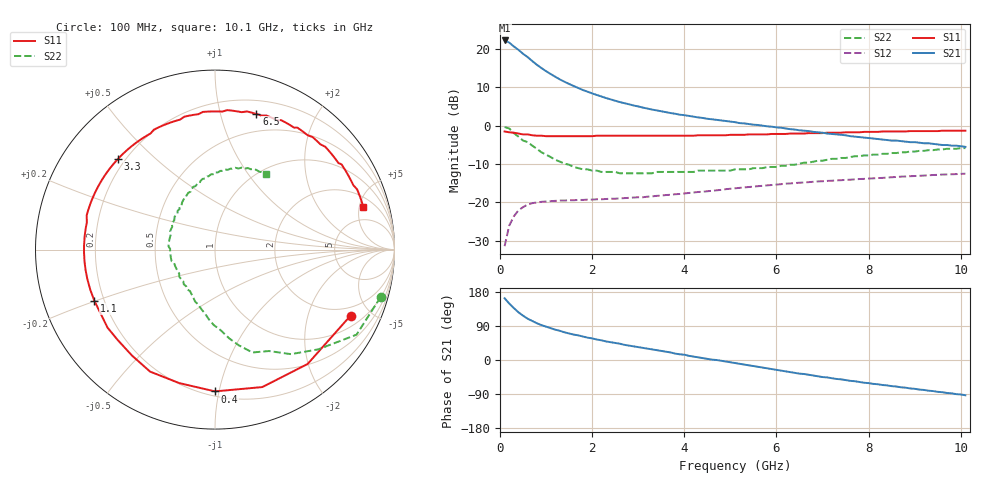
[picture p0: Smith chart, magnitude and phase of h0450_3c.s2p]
!HBFP-0450
!S and NOISE PARAMETERS at Vce=3V  Ic=5mA.  LAST UPDATED  09-04-98
# GHZ S MA R  50
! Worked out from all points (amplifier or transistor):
!   101 points, 100 MHz to 10.1 GHz, reference 50 ohm
!   highest |S21| = 22.2 dB at 100 MHz (marker M1)
!   |S21| within 3 dB of that: start of sweep to 454.6 MHz
!   unconditionally stable (mu >= 1): 2.917 GHz to end of sweep
!   at 1.7 GHz: K = 0.62, MSG = 14.6 dB, |S12| = -19.3 dB
!   at 5.1 GHz: K = 1.23, MAG = 5.7 dB, |S12| = -16.3 dB
!   at 10.1 GHz: K = 1.12, MAG = 1.4 dB, |S12| = -12.5 dB
!   lowest NFmin = 1.14 dB at 1.8 GHz
!   S11 on the Smith chart (normalised r, x): 100 MHz: 1.50, -3.76; 400 MHz: 0.23, -0.97; 1.1 GHz: 0.16, -0.20; 3.3 GHz: 0.17, +0.38; 6.5 GHz: 0.32, +1.30; 10.1 GHz: 3.02, +5.50
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0.1  0.84 -26.0  12.86 163.0  0.027 75.0  0.96 -16.0
0.2  0.82 -51.0  12.07 149.0  0.05 62.0  0.92 -31.0
0.3  0.81 -71.0  10.74 137.0  0.066 52.0  0.8 -44.0
0.4  0.79 -90.0  9.71 126.0  0.079 44.0  0.72 -54.0
0.5  0.77 -105.0  8.63 117.0  0.087 38.0  0.64 -62.0
0.6  0.77 -118.0  7.81 109.0  0.094 32.0  0.61 -70.0
0.7  0.75 -128.0  6.94 103.0  0.098 28.0  0.55 -76.0
0.8  0.74 -137.0  6.2 97.0  0.1 25.0  0.5 -81.0
0.9  0.74 -144.0  5.62 92.0  0.102 22.0  0.45 -86.0
1.1  0.73 -157.0  4.7 84.0  0.104 18.0  0.39 -95.0
1.4  0.73 -171.0  3.73 73.0  0.106 14.0  0.32 -107.0
1.8  0.73 174.0  2.91 62.0  0.108 11.0  0.27 -121.0
2.3  0.74 160.0  2.29 49.0  0.111 8.0  0.25 -138.0
2.7  0.74 150.0  1.96 40.0  0.114 7.0  0.24 -149.0
3.3  0.74 137.0  1.62 28.0  0.12 5.0  0.24 -163.0
3.5  0.74 133.0  1.54 24.0  0.123 4.0  0.25 -167.0
4.3  0.75 117.0  1.28 7.0  0.137 1.0  0.26 176.0
5.1  0.76 101.0  1.11 -8.0  0.153 -5.0  0.27 158.0
6.5  0.79 73.0  0.87 -36.0  0.181 -19.0  0.32 125.0
6.8  0.8 68.0  0.83 -41.0  0.186 -22.0  0.34 118.0
8.5  0.84 40.0  0.64 -69.0  0.213 -42.0  0.44 86.0
10.1  0.86 16.0  0.53 -93.0  0.237 -63.0  0.51 56.0
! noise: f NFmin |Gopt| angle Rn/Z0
1.8  1.14  0.53  165  0.04
2  1.21  0.53  172  0.04
2.5  1.4  0.56  -170  0.05
3.5  1.74  0.66  -143  0.14
4  1.98  0.68  -129  0.27
5  2.34  0.71  -106  0.69
5.5  2.56  0.75  -95  1.02
7  3.09  0.8  -64  2.46
8  3.5  0.82  -47  3.82
10  4.2  0.83  -16  6.44
